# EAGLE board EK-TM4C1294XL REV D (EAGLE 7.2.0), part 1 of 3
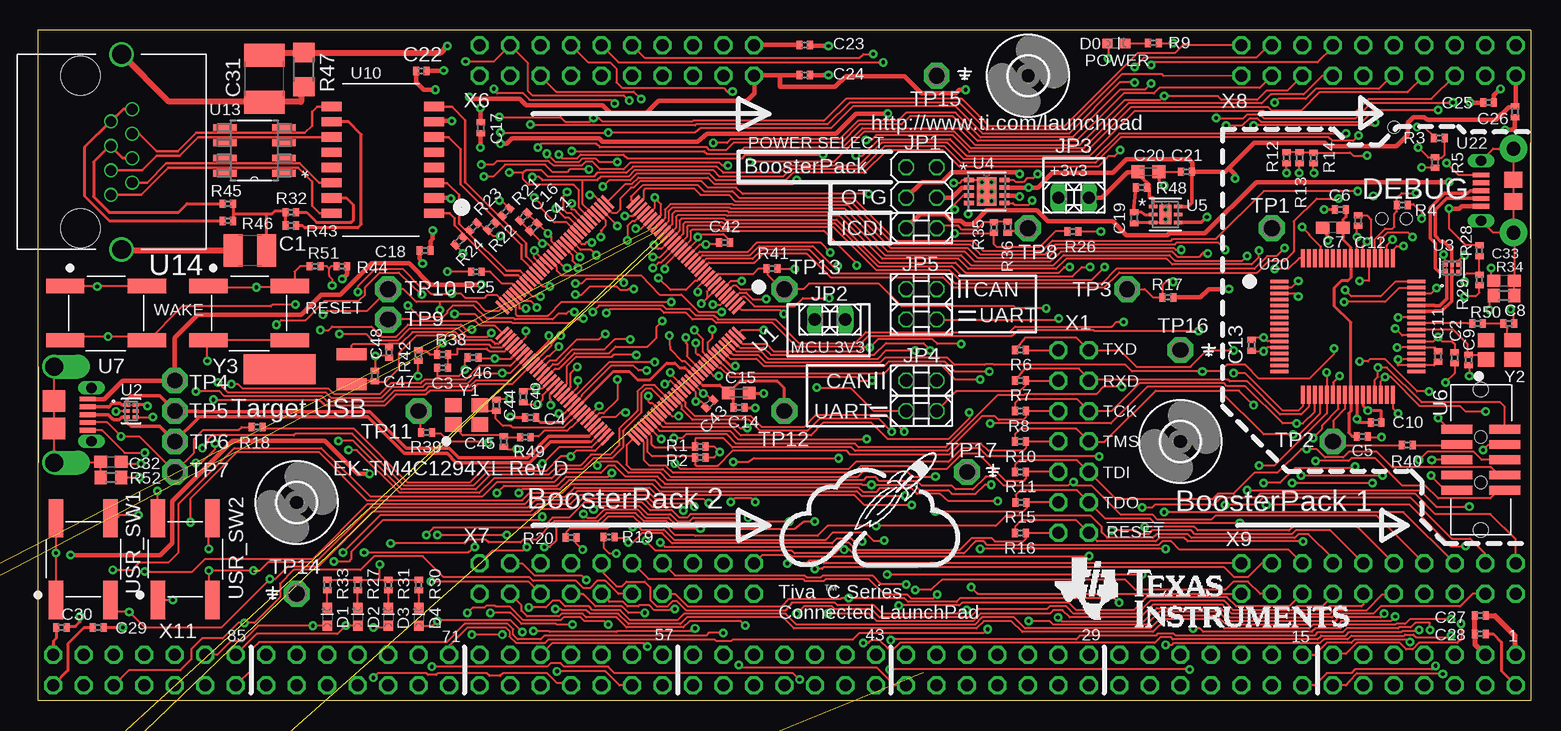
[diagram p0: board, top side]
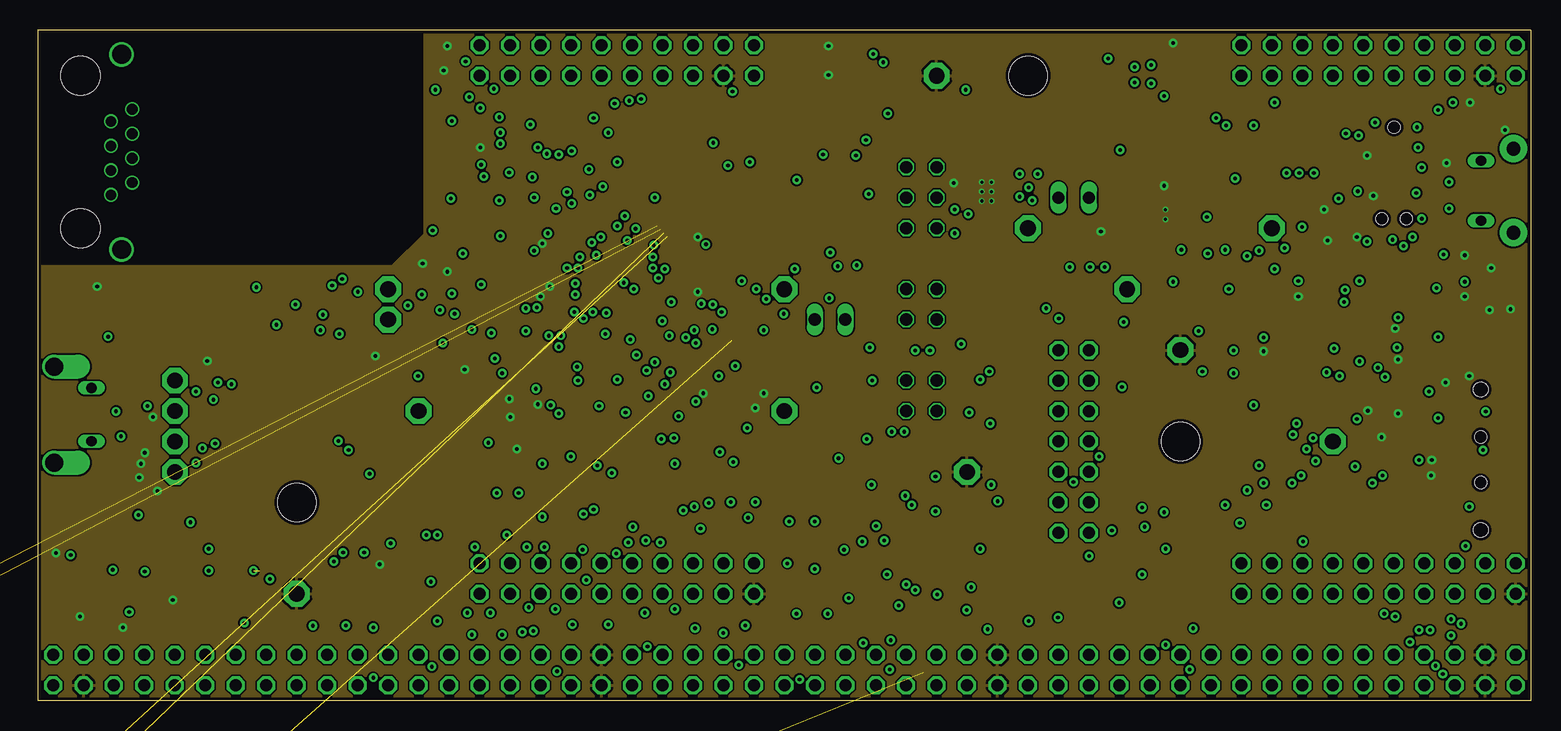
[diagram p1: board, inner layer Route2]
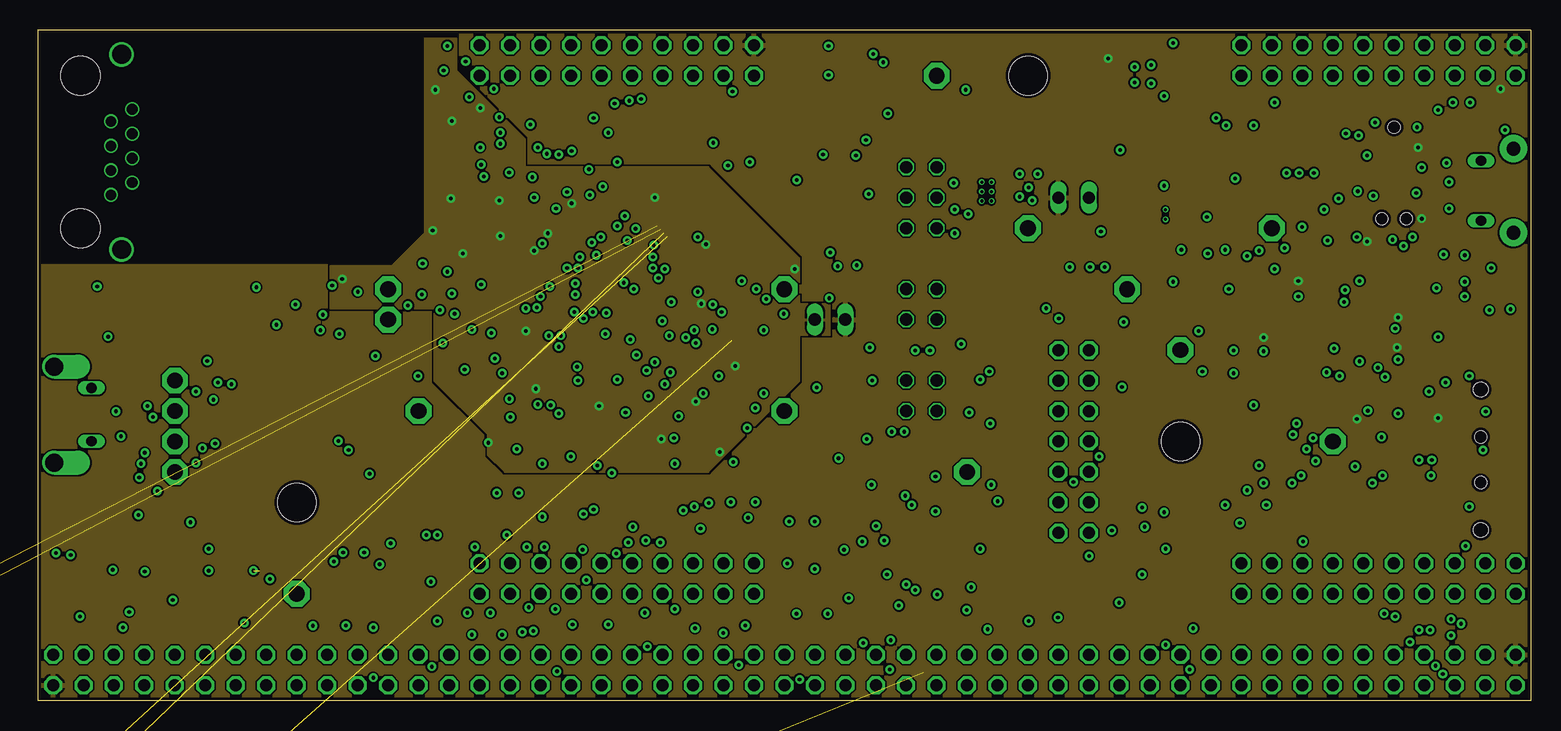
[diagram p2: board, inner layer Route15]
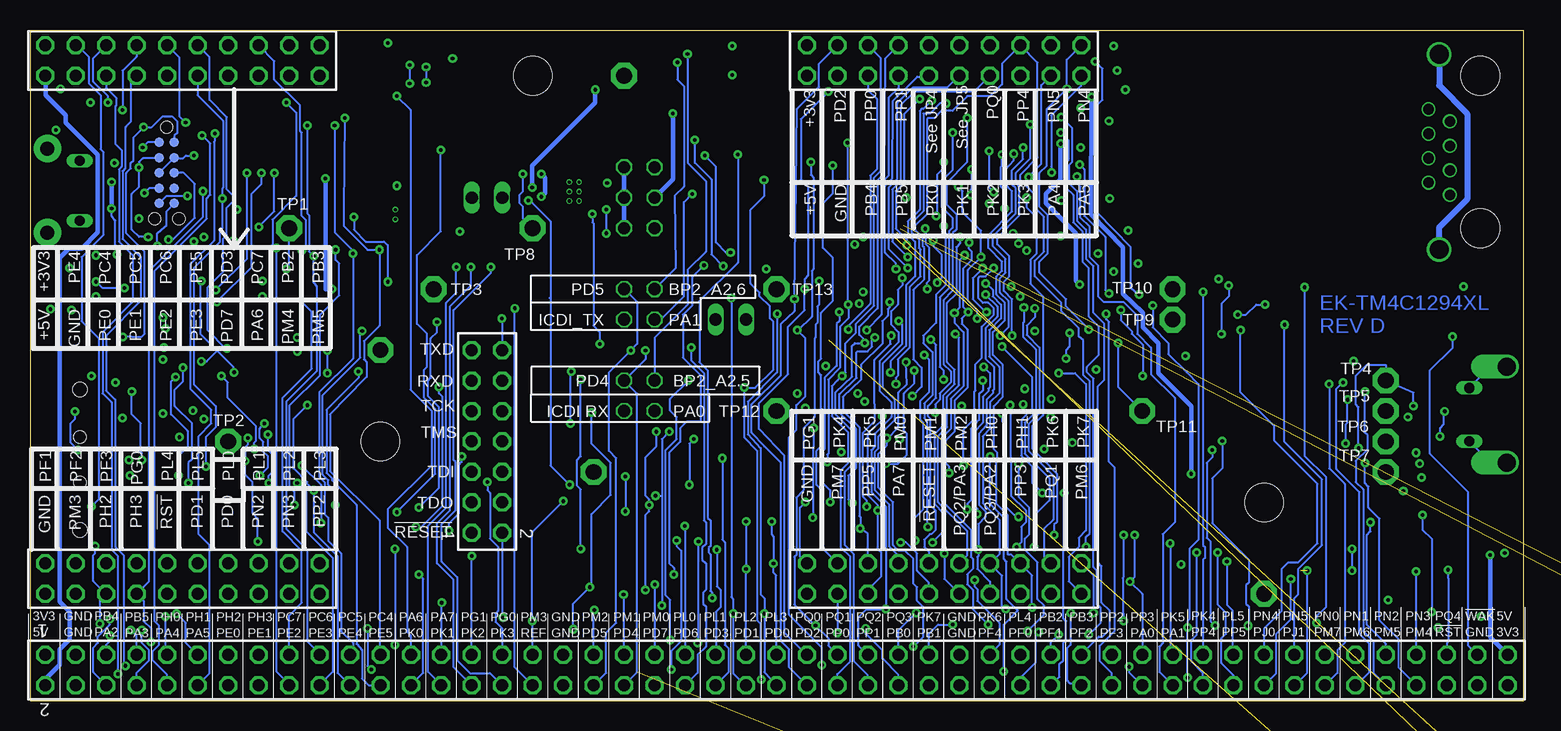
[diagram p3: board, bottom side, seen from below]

Size 124.46 x 55.88 mm. Coordinates in mm from the lower left corner, seen from the top.
Outline: 124.46,55.88 124.46,0 0,0 0,55.88 124.46,55.88
Copper layers (1+2*15+16): Top 0.035mm / dielectric 0.22mm / Route2 0.035mm / dielectric 1mm / Route15 0.035mm / dielectric 0.22mm / Bottom 0.035mm
Design rules "default *": minimum track width 6mil, minimum drill 12mil, track to track 6mil, track to pad 6mil, pad to pad 5mil, via to via 6mil, smd to smd 5mil, copper to edge 10mil, drill to drill 8mil, minimum pad ring 4mil, minimum via ring 8mil, stop-mask expansion 2mil, vias tented up to drill 13mil, thermal gap 8mil
Net classes: 1 USB: width 0.275 mm, clearance 0.152 mm; 2 Ethernet: width 0.22 mm, clearance 0.152 mm

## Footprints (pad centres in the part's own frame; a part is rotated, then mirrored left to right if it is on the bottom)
C1210 = smd 1.6 x 2.7: 1 -1.4,0; 2 1.4,0
C0402 = smd 0.5 x 0.7: 1 -0.45,0; 2 0.45,0
C0603 = smd 1.1 x 1: 1 -0.85,0; 2 0.85,0
C0603K = smd 1.05 x 1.08: 1 -0.875,0; 2 0.875,0
C1812 = smd 1.9 x 3.4: 1 -1.95,0; 2 1.95,0
CHIPLED_0603 = smd 0.8 x 0.8: A 0,-0.75; C 0,0.75
3,2 = hole 3.2: 0,0
2X03 = drill 1.016 octagon: 1 -2.54,-1.27; 2 -2.54,1.27; 3 0,-1.27; 4 0,1.27; 5 2.54,-1.27; 6 2.54,1.27
1X02 = drill 1.016 long: 1 -1.27,0; 2 1.27,0
2X02 = drill 1.016 octagon: 1 -1.27,-1.27; 2 -1.27,1.27; 3 1.27,-1.27; 4 1.27,1.27
R0402 = smd 0.5 x 0.7: 1 -0.45,0; 2 0.45,0
R0603 = smd 1 x 1.1: 1 -0.85,0; 2 0.85,0
R1206 = smd 1.6 x 1.803: 1 -1.422,0; 2 1.422,0
SWITCH_6MM_6MM_TE_CON_SMD = smd 1.2 x 3.2: P$1 4.521,6.807; P$2 4.521,0; P$3 0,6.807; P$4 0,0
P1-13 = drill 1.321 pad 2.159 octagon: TP 0,0
TQFP-128 = smd 1.45 x 0.25: P$1 0,0; P$2 0,-0.4; P$3 0,-0.8; P$4 0,-1.2; P$5 0,-1.6; P$6 0,-2; P$7 0,-2.4; P$8 0,-2.8; P$9 0,-3.2; P$10 0,-3.6; P$11 0,-4; P$12 0,-4.4; P$13 0,-4.8; P$14 0,-5.2; P$15 0,-5.6; P$16 0,-6; P$17 0,-6.4; P$18 0,-6.8; P$19 0,-7.2; P$20 0,-7.6; P$21 0,-8; P$22 0,-8.4; P$23 0,-8.8; P$24 0,-9.2; P$25 0,-9.6; P$26 0,-10; P$27 0,-10.4; P$28 0,-10.8; P$29 0,-11.2; P$30 0,-11.6; P$31 0,-12; P$32 0,-12.4; P$65 15.45,-12.4; P$66 15.45,-12; P$67 15.45,-11.6; P$68 15.45,-11.2; P$69 15.45,-10.8; P$70 15.45,-10.4; P$71 15.45,-10; P$72 15.45,-9.6; P$73 15.45,-9.2; P$74 15.45,-8.8; P$75 15.45,-8.4; P$76 15.45,-8; P$77 15.45,-7.6; P$78 15.45,-7.2; P$79 15.45,-6.8; P$80 15.45,-6.4; P$81 15.45,-6; P$82 15.45,-5.6; P$83 15.45,-5.2; P$84 15.45,-4.8; P$85 15.45,-4.4; P$86 15.45,-4; P$87 15.45,-3.6; P$88 15.45,-3.2; P$89 15.45,-2.8; P$90 15.45,-2.4; P$91 15.45,-2; P$92 15.45,-1.6; P$93 15.45,-1.2; P$94 15.45,-0.8; P$95 15.45,-0.4; P$96 15.45,0 | smd 0.25 x 1.45: P$33 1.525,-13.925; P$34 1.925,-13.925; P$35 2.325,-13.925; P$36 2.725,-13.925; P$37 3.125,-13.925; P$38 3.525,-13.925; P$39 3.925,-13.925; P$40 4.325,-13.925; P$41 4.725,-13.925; P$42 5.125,-13.925; P$43 5.525,-13.925; P$44 5.925,-13.925; P$45 6.325,-13.925; P$46 6.725,-13.925; P$47 7.125,-13.925; P$48 7.525,-13.925; P$49 7.925,-13.925; P$50 8.325,-13.925; P$51 8.725,-13.925; P$52 9.125,-13.925; P$53 9.525,-13.925; P$54 9.925,-13.925; P$55 10.325,-13.925; P$56 10.725,-13.925; P$57 11.125,-13.925; P$58 11.525,-13.925; P$59 11.925,-13.925; P$60 12.325,-13.925; P$61 12.725,-13.925; P$62 13.125,-13.925; P$63 13.525,-13.925; P$64 13.925,-13.925; P$97 13.925,1.525; P$98 13.525,1.525; P$99 13.125,1.525; P$100 12.725,1.525; P$101 12.325,1.525; P$102 11.925,1.525; P$103 11.525,1.525; P$104 11.125,1.525; P$105 10.725,1.525; P$106 10.325,1.525; P$107 9.925,1.525; P$108 9.525,1.525; P$109 9.125,1.525; P$110 8.725,1.525; P$111 8.325,1.525; P$112 7.925,1.525; P$113 7.525,1.525; P$114 7.125,1.525; P$115 6.725,1.525; P$116 6.325,1.525; P$117 5.925,1.525; P$118 5.525,1.525; P$119 5.125,1.525; P$120 4.725,1.525; P$121 4.325,1.525; P$122 3.925,1.525; P$123 3.525,1.525; P$124 3.125,1.525; P$125 2.725,1.525; P$126 2.325,1.525; P$127 1.925,1.525; P$128 1.525,1.525
DRY6 = smd 0.559 x 0.305: 1 -0.356,0.508 | smd 0.508 x 0.305: 2 -0.381,0; 3 -0.381,-0.508; 4 0.381,-0.508; 5 0.381,0; 6 0.381,0.508
DRB8_2P4X1P65 = smd 0.838 x 0.356: 1 -1.473,0.965; 2 -1.473,0.33; 3 -1.473,-0.33; 4 -1.473,-0.965; 5 1.473,-0.965; 6 1.473,-0.33; 7 1.473,0.33; 8 1.473,0.965 | smd 1.651 x 2.388: 9 0,0 | drill 0.254: V 0.406,0.787; V_2 -0.406,0; V_3 -0.406,-0.787; V_4 -0.406,0.787; V_5 0.406,-0.787; V_6 0.406,0
DRV6_1P6X1 = smd 0.711 x 0.305: 1 -1.041,0.66; 2 -1.041,0; 3 -1.041,-0.66; 4 1.041,-0.66; 5 1.041,0; 6 1.041,0.66 | smd 1.016 x 1.6: 7 0,0 | drill 0.254: V 0,-0.406; V_2 0,0.406
CON_2X5_50MIL = smd 0.74 x 2.6: P1 0,0; P2 0,4.008; P3 1.27,0; P4 1.27,4.008; P5 2.54,0; P6 2.54,4.008; P7 3.81,0; P8 3.81,4.008; P9 5.08,0; P10 5.08,4.008 | hole 1: 4.44,2; 0.64,2 | hole 1.2: 8.407,2; -3.327,2
CON_USB_MICRO_AB_HIROSE_ZX62D-AB-5P8 = smd 1.35 x 0.4: P1 2.8,1.3; P2 2.8,0.65; P3 2.8,0; P4 2.8,-0.65; P5 2.8,-1.3 | smd 1.9 x 1.8: P$1 0,-1.15; P$2 0,1.15 | drill 0.85 pad 1.092 long: P$3 3.125,2.225; P$4 3.125,-2.225 | drill 1.5 pad 2 offset: P$5 0,-4; P$6 0,4
DIL28-3 = drill 0.813 long: 1 -16.51,-3.81; 2 -13.97,-3.81; 3 -11.43,-3.81; 4 -8.89,-3.81; 5 -6.35,-3.81; 6 -3.81,-3.81; 7 -1.27,-3.81; 8 1.27,-3.81; 9 3.81,-3.81; 10 6.35,-3.81; 11 8.89,-3.81; 12 11.43,-3.81; 13 13.97,-3.81; 14 16.51,-3.81; 15 16.51,3.81; 16 13.97,3.81; 17 11.43,3.81; 18 8.89,3.81; 19 6.35,3.81; 20 3.81,3.81; 21 1.27,3.81; 22 -1.27,3.81; 23 -3.81,3.81; 24 -6.35,3.81; 25 -8.89,3.81; 26 -11.43,3.81; 27 -13.97,3.81; 28 -16.51,3.81
MAG_PULSE_HX1188FNL = smd 0.76 x 1.67: P$1 0,0; P$2 1.27,0; P$3 2.54,0; P$4 3.81,0; P$5 5.08,0; P$6 6.35,0; P$7 7.62,0; P$8 8.89,0; P$9 8.89,8.55; P$10 7.62,8.55; P$11 6.35,8.55; P$12 5.08,8.55; P$13 3.81,8.55; P$14 2.54,8.55; P$15 1.27,8.55; P$16 0,8.55
BLUETOOTH_SMD = smd 2 x 1: 1 0,0; 2 0,-1.5; 3 0,-3; 4 0,-4.5; 5 0,-6; 6 0,-7.5; 7 0,-9; 8 0,-10.5; 9 0,-12; 10 0,-13.5; 11 0,-15; 12 0,-16.5; 13 0,-18; 22 13,-18; 23 13,-16.5; 24 13,-15; 25 13,-13.5; 26 13,-12; 27 13,-10.5; 28 13,-9; 29 13,-7.5; 30 13,-6; 31 13,-4.5; 32 13,-3; 33 13,-1.5; 34 13,0 | smd 1 x 1.8: 14 1.25,-19.75; 15 2.75,-19.75; 16 4.25,-19.75; 17 5.75,-19.75; 18 7.25,-19.75; 19 8.75,-19.75; 20 10.25,-19.75; 21 11.75,-19.75
D8 = smd 1.981 x 0.559: 1 -2.464,1.905; 2 -2.464,0.635; 3 -2.464,-0.635; 4 -2.464,-1.905; 5 2.464,-1.905; 6 2.464,-0.635; 7 2.464,0.635; 8 2.464,1.905
RJ45_TE_CON_NOMAG_NOLED = drill 0.89: 1 9.93,2.54; 2 8.91,4.32; 3 7.89,2.54; 4 6.87,4.32; 5 5.85,2.54; 6 4.83,4.32; 7 3.81,2.54; 8 2.79,4.32 | drill 1.57: 9 -1.78,3.43; 10 14.48,3.43 | hole 3.25: 0,0; 12.7,0
LQFP-64-PM = smd 1.5 x 0.3: P$1 0,0; P$2 0,-0.5; P$3 0,-1; P$4 0,-1.5; P$5 0,-2; P$6 0,-2.5; P$7 0,-3; P$8 0,-3.5; P$9 0,-4; P$10 0,-4.5; P$11 0,-5; P$12 0,-5.5; P$13 0,-6; P$14 0,-6.5; P$15 0,-7; P$16 0,-7.5; P$33 11.4,-7.5; P$34 11.4,-7; P$35 11.4,-6.5; P$36 11.4,-6; P$37 11.4,-5.5; P$38 11.4,-5; P$39 11.4,-4.5; P$40 11.4,-4; P$41 11.4,-3.5; P$42 11.4,-3; P$43 11.4,-2.5; P$44 11.4,-2; P$45 11.4,-1.5; P$46 11.4,-1; P$47 11.4,-0.5; P$48 11.4,0 | smd 0.3 x 1.5: P$17 1.95,-9.45; P$18 2.45,-9.45; P$19 2.95,-9.45; P$20 3.45,-9.45; P$21 3.95,-9.45; P$22 4.45,-9.45; P$23 4.95,-9.45; P$24 5.45,-9.45; P$25 5.95,-9.45; P$26 6.45,-9.45; P$27 6.95,-9.45; P$28 7.45,-9.45; P$29 7.95,-9.45; P$30 8.45,-9.45; P$31 8.95,-9.45; P$32 9.45,-9.45; P$49 9.45,1.95; P$50 8.95,1.95; P$51 8.45,1.95; P$52 7.95,1.95; P$53 7.45,1.95; P$54 6.95,1.95; P$55 6.45,1.95; P$56 5.95,1.95; P$57 5.45,1.95; P$58 4.95,1.95; P$59 4.45,1.95; P$60 3.95,1.95; P$61 3.45,1.95; P$62 2.95,1.95; P$63 2.45,1.95; P$64 1.95,1.95
TC2030-MCP-NL = smd 0.787 x 0.787: 1 1.27,-0.635; 2 2.54,-0.635; 3 3.81,-0.635; 4 5.08,-0.635; 5 6.35,-0.635; 6 6.35,0.635; 7 5.08,0.635; 8 3.81,0.635; 9 2.54,0.635; 10 1.27,0.635 | hole 1: 0,0; 7.62,-1.016; 7.62,1.016
CON_USB_MICRO_B_FCI_10118194 = smd 1.35 x 0.4: P1 2.7,1.3; P2 2.7,0.65; P3 2.7,0; P4 2.7,-0.65; P5 2.7,-1.3 | smd 1.5 x 1.35: P6 0,0.9; P7 0,-0.9 | drill 0.85 long: P8 2.7,2.5; P9 2.7,-2.5 | drill 1.15 pad 2.286: P10 0,-3.5; P11 0,3.5
TSW-107-02-S-D = drill 1 pad 1.5 octagon: 1 7.62,-1.27; 2 7.62,1.27; 3 5.08,-1.27; 4 5.08,1.27; 5 2.54,-1.27; 6 2.54,1.27; 7 0,-1.27; 8 0,1.27; 9 -2.54,-1.27; 10 -2.54,1.27; 11 -5.08,-1.27; 12 -5.08,1.27; 13 -7.62,-1.27; 14 -7.62,1.27
TSW-110-02-S-D = drill 1 pad 1.5 octagon: 1 11.43,-1.27; 2 11.43,1.27; 3 8.89,-1.27; 4 8.89,1.27; 5 6.35,-1.27; 6 6.35,1.27; 7 3.81,-1.27; 8 3.81,1.27; 9 1.27,-1.27; 10 1.27,1.27; 11 -1.27,-1.27; 12 -1.27,1.27; 13 -3.81,-1.27; 14 -3.81,1.27; 15 -6.35,-1.27; 16 -6.35,1.27; 17 -8.89,-1.27; 18 -8.89,1.27; 19 -11.43,-1.27; 20 -11.43,1.27
TSW-149-02-S-D = drill 1 pad 1.5 octagon: 1 60.96,-1.27; 2 60.96,1.27; 3 58.42,-1.27; 4 58.42,1.27; 5 55.88,-1.27; 6 55.88,1.27; 7 53.34,-1.27; 8 53.34,1.27; 9 50.8,-1.27; 10 50.8,1.27; 11 48.26,-1.27; 12 48.26,1.27; 13 45.72,-1.27; 14 45.72,1.27; 15 43.18,-1.27; 16 43.18,1.27; 17 40.64,-1.27; 18 40.64,1.27; 19 38.1,-1.27; 20 38.1,1.27; 21 35.56,-1.27; 22 35.56,1.27; 23 33.02,-1.27; 24 33.02,1.27; 25 30.48,-1.27; 26 30.48,1.27; 27 27.94,-1.27; 28 27.94,1.27; 29 25.4,-1.27; 30 25.4,1.27; 31 22.86,-1.27; 32 22.86,1.27; 33 20.32,-1.27; 34 20.32,1.27; 35 17.78,-1.27; 36 17.78,1.27; 37 15.24,-1.27; 38 15.24,1.27; 39 12.7,-1.27; 40 12.7,1.27; 41 10.16,-1.27; 42 10.16,1.27; 43 7.62,-1.27; 44 7.62,1.27; 45 5.08,-1.27; 46 5.08,1.27; 47 2.54,-1.27; 48 2.54,1.27; 49 0,-1.27; 50 0,1.27; 51 -2.54,-1.27; 52 -2.54,1.27; 53 -5.08,-1.27; 54 -5.08,1.27; 55 -7.62,-1.27; 56 -7.62,1.27; 57 -10.16,-1.27; 58 -10.16,1.27; 59 -12.7,-1.27; 60 -12.7,1.27; 61 -15.24,-1.27; 62 -15.24,1.27; 63 -17.78,-1.27; 64 -17.78,1.27; 65 -20.32,-1.27; 66 -20.32,1.27; 67 -22.86,-1.27; 68 -22.86,1.27; 69 -25.4,-1.27; 70 -25.4,1.27; 71 -27.94,-1.27; 72 -27.94,1.27; 73 -30.48,-1.27; 74 -30.48,1.27; 75 -33.02,-1.27; 76 -33.02,1.27; 77 -35.56,-1.27; 78 -35.56,1.27; 79 -38.1,-1.27; 80 -38.1,1.27; 81 -40.64,-1.27; 82 -40.64,1.27; 83 -43.18,-1.27; 84 -43.18,1.27; 85 -45.72,-1.27; 86 -45.72,1.27; 87 -48.26,-1.27; 88 -48.26,1.27; 89 -50.8,-1.27; 90 -50.8,1.27; 91 -53.34,-1.27; 92 -53.34,1.27; 93 -55.88,-1.27; 94 -55.88,1.27; 95 -58.42,-1.27; 96 -58.42,1.27; 97 -60.96,-1.27; 98 -60.96,1.27
NDK3.2X2.5 = smd 1.4 x 1.2: P$1 0,0; P$2 2.2,0; P$3 2.2,1.6; P$4 0,1.6
CRYSTAL_32K_SMD = smd 2.5 x 1: P$1 0,1.25; P$2 0,-1.25 | smd 6 x 2.5: P$3 -6,0

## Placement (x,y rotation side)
C1  1000pF  [C1210]  17.68,37.49 180 top
C2  0.1uF  [C0402]  118.11,28.57 270 top
C3  0.1uF  [C0402]  33.76,27.74 180 top
C4  0.1uF  [C0402]  41.07,23.6 180 top
C5  0.1uF  [C0402]  110.41,22 0 top
C6  1.0uF  [C0402]  108.58,40.92 180 top
C7  2.2uF  [C0603]  107.95,39.42 180 top
C8  12pF  [C0402]  122.63,31.42 0 top
C9  12pF  [C0402]  119.25,28.37 270 top
C10  0.1uF  [C0402]  111.56,23.16 0 top
C11  0.1uF  [C0402]  116.71,28.68 270 top
C12  0.1uF  [C0402]  110.06,40.01 270 top
C13  0.1uF  [C0402]  101.17,29.62 270 top
C14  1.0uF  [C0402]  58.45,24.41 0 top
C15  2.2uF  [C0603K]  58.45,25.63 0 top
C16  0.1uF  [C0402]  40.49,40.31 225 top
C17  0.1uF  [C0402]  36.93,47.73 270 top
C18  0.1uF  [C0402]  32.28,37.49 180 top
C19  0.1uF  [C0402]  91.39,40.23 270 top
C20  2.2uF  [C0603K]  92.58,44.07 0 top
C21  0.1uF  [C0402]  95.76,44.07 180 top
C22  0.1uF  [C0402]  31.98,52.48 0 top
C23  0.1uF  [C0402]  63.93,54.64 0 top
C24  0.1uF  [C0402]  63.93,52.12 0 top
C25  0.1uF  [C0402]  120.93,49.83 180 top
C26  0.1uF  [C0402]  123.14,49.07 270 top
C27  0.1uF  [C0402]  120.24,7.09 180 top
C28  0.1uF  [C0402]  120.24,5.56 180 top
C29  0.1uF  [C0402]  5.03,6.1 0 top
C30  0.1uF  [C0402]  1.98,6.1 0 top
C31  4700pF  [C1812]  18.9,51.82 90 top
C32  3300pF  [C0603]  6.1,19.89 0 top
C33  3300pF  [C0603]  122.22,34.98 180 top
C40  0.1uF  [C0402]  40.46,25.32 270 top
C41  0.1uF  [C0402]  41.33,39.45 225 top
C42  0.1uF  [C0402]  57.25,38.18 0 top
C43  0.1uF  [C0402]  56.01,24.74 45 top
C44  12pF  [C0402]  38.23,24.61 90 top
C45  12pF  [C0402]  38.84,21.59 270 top
C46  0.1uF  [C0402]  36.3,28.6 180 top
C47  12pF  [C0402]  28.09,27.05 90 top
C48  12pF  [C0402]  29.29,29.01 270 top
D0  [CHIPLED_0603]  89.92,54.76 270 top
D1  [CHIPLED_0603]  24.13,6.99 0 top
D2  [CHIPLED_0603]  26.67,6.99 0 top
D3  [CHIPLED_0603]  29.21,6.99 0 top
D4  [CHIPLED_0603]  31.75,6.99 0 top
H1  MOUNT-HOLE3.2  [3,2]  95.25,21.59 0 top
H4  MOUNT-HOLE3.2  [3,2]  21.59,16.51 0 top
H6  MOUNT-HOLE3.2  [3,2]  82.55,52.07 0 top
J1  [JUMP]  73.66,39.37 90 top
J2  [JUMP]  73.66,24.13 90 top
J3  [JUMP]  86.36,41.91 90 top
J4  [JUMP]  73.66,26.67 90 top
J5  [JUMP]  73.66,31.75 90 top
J6  [JUMP]  73.66,34.29 90 top
J7  [JUMP]  66.04,31.75 90 top
JP1  [2X03]  73.66,41.91 270 top
JP2  [1X02]  66.04,31.75 180 top
JP3  [1X02]  86.36,41.91 0 top
JP4  [2X02]  73.66,25.4 90 top
JP5  [2X02]  73.66,33.02 90 top
R1  10k  [R0402]  55.22,21.18 180 top
R2  10k  [R0402]  55.22,20.24 180 top
R3  10k  [R0402]  116.84,46.89 0 top
R4  10k  [R0402]  113.74,41.3 180 top
R5  10k  [R0402]  116.48,44.83 270 top
R6  0  [R0402]  81.92,29.21 180 top
R7  0  [R0402]  81.92,26.67 180 top
R8  0  [R0402]  81.92,24.13 180 top
R9  330  [R0402]  92.99,54.81 180 top
R10  0  [R0402]  81.92,21.59 180 top
R11  0  [R0402]  81.92,19.05 180 top
R12  5.6k  [R0402]  104.09,45.24 90 top
R13  5.6k  [R0402]  105.18,45.24 90 top
R14  5.6k  [R0402]  106.35,45.21 90 top
R15  0  [R0402]  81.97,16.51 180 top
R16  0  [R0402]  81.92,13.97 180 top
R17  100k  [R0402]  94.21,33.6 180 top
R18  100  [R0402]  18.29,22.78 180 top
R19  0  [R0402]  47.62,13.61 0 top
R20  0  [R0402]  44.45,13.59 180 top
R21  49.9  [R0402]  39.01,40.72 225 top
R22  49.9  [R0402]  37.82,39.52 45 top
R23  49.4  [R0402]  36.3,39.47 225 top
R24  49.9  [R0402]  35.1,38.28 45 top
R25  4.87k 1%  [R0402]  36.55,35.74 180 top
R26  100k  [R0402]  86.28,39.09 0 top
R27  330  [R0402]  26.67,9.63 270 top
R28  5.6k  [R0402]  120.17,37.49 90 top
R29  10k  [R0402]  120.17,35.05 90 top
R30  330  [R0402]  31.75,9.63 270 top
R31  330  [R0402]  29.21,9.63 270 top
R32  75  [R0402]  21.11,40.69 0 top
R33  330  [R0402]  24.13,9.63 270 top
R34  1M  [R0603]  122.22,33.76 0 top
R35  10k  [R0402]  79.71,39.42 270 top
R36  100k  [R0402]  80.85,39.45 90 top
R38  51  [R0402]  33.76,28.83 0 top
R39  0  [R0402]  32.41,22.33 0 top
R40  0  [R0402]  114.17,21.29 0 top
R41  0  [R0402]  61.21,36.02 0 top
R42  1M  [R0402]  31.72,28.75 270 top
R43  75  [R0402]  21.11,39.57 0 top
R44  10k  [R0402]  25.35,36.2 180 top
R45  75  [R0402]  15.85,41.4 180 top
R46  75  [R0402]  15.85,39.98 180 top
R47  1M  [R1206]  22.17,52.58 270 top
R48  [R0402]  92,42.76 0 top
R49  2k  [R0402]  40.64,21.95 0 top
R50  2k  [R0402]  120.02,31.42 0 top
R51  100  [R0402]  23.13,36.2 0 top
R52  1M  [R0603]  6.1,18.59 180 top
RESET  SWITCH_TACTILE  [SWITCH_6MM_6MM_TE_CON_SMD]  14.22,34.54 270 top
TP1  TPPAD1-13  [P1-13]  102.87,39.37 270 top
TP2  TPPAD1-13  [P1-13]  107.95,21.59 0 top
TP3  TPPAD1-13  [P1-13]  90.81,34.29 180 top
TP4  TPPAD1-13  [P1-13]  11.43,26.67 90 top
TP5  TPPAD1-13  [P1-13]  11.43,24.13 270 top
TP6  TPPAD1-13  [P1-13]  11.43,21.59 90 top
TP7  TPPAD1-13  [P1-13]  11.43,19.05 270 top
TP8  TPPAD1-13  [P1-13]  82.55,39.37 180 top
TP9  TPPAD1-13  [P1-13]  29.21,31.75 0 top
TP10  TPPAD1-13  [P1-13]  29.21,34.29 0 top
TP11  TPPAD1-13  [P1-13]  31.75,24.13 0 top
TP12  TPPAD1-13  [P1-13]  62.23,24.13 0 top
TP13  TPPAD1-13  [P1-13]  62.23,34.29 0 top
TP14  TPPAD1-13  [P1-13]  21.59,8.89 0 top
TP15  TPPAD1-13  [P1-13]  74.93,52.07 0 top
TP16  TPPAD1-13  [P1-13]  95.25,29.21 0 top
TP17  TPPAD1-13  [P1-13]  77.47,19.05 0 top
U1  TM4C1294NCPDT  [TQFP-128]  58.42,32.77 225 top
U2  TPD4S012_DRY_6  [DRY6]  7.77,24.13 0 top
U3  TPD4S012_DRY_6  [DRY6]  117.88,36.04 90 top
U4  TPS2052B_DRB_8  [DRB8_2P4X1P65]  79.1,42.42 0 top
U5  TPS73733_DRV_6  [DRV6_1P6X1]  94,40.5 0 top
U6  JTAG_ARM_10PIN  [CON_2X5_50MIL]  118.29,22.61 270 top
U7  CON_USB_HIROSE_MICRO_AB_ZX62D_AB_5P8  [CON_USB_MICRO_AB_HIROSE_ZX62D-AB-5P8]  1.35,23.83 0 top
U8  ATMEGA328P_PDIP  [DIL28-3]  not placed on the board
U9  ATMEGA328P_PDIP  [DIL28-3]  not placed on the board
U10  MAG_PULSE_HX1188FNL  [MAG_PULSE_HX1188FNL]  33.05,40.61 90 top
U11  HC_05  [BLUETOOTH_SMD]  not placed on the board
U13  SLVU2.8-4  [D8]  18.06,45.85 180 top
U14  JACK_RJ45_NOMAG_NOLED_TECON  [RJ45_TE_CON_NOMAG_NOLED]  3.56,52.07 270 top
U20  TM4C123GH6PMI  [LQFP-64-PM]  103.5,34.92 0 top
U21  TC2050-NL-MCP-NL  [TC2030-MCP-NL]  113.06,47.78 270 bottom
U22  CON_USB_FCI_MICRO_B_10118194  [CON_USB_MICRO_B_FCI_10118194]  123.01,42.49 180 top
USR_SW1  SWITCH_TACTILE  [SWITCH_6MM_6MM_TE_CON_SMD]  1.52,8.38 0 top
USR_SW2  SWITCH_TACTILE  [SWITCH_6MM_6MM_TE_CON_SMD]  10.03,8.38 0 top
WAKE  SWITCH_TACTILE  [SWITCH_6MM_6MM_TE_CON_SMD]  2.29,34.54 270 top
X1  TSW-107-02-S-D  [TSW-107-02-S-D]  86.36,21.59 270 bottom
X6  TSW-110-02-S-D  [TSW-110-02-S-D]  48.26,53.34 180 bottom
X7  TSW-110-02-S-D  [TSW-110-02-S-D]  48.26,10.16 180 bottom
X8  TSW-110-02-S-D  [TSW-110-02-S-D]  111.76,53.34 180 bottom
X9  TSW-110-02-S-D  [TSW-110-02-S-D]  111.76,10.16 180 bottom
X11  TSW-149-02-S-D  [TSW-149-02-S-D]  62.23,2.54 180 bottom
Y1  25Mhz  [NDK3.2X2.5]  34.65,23.01 0 top
Y2  16M  [NDK3.2X2.5]  120.73,28.42 0 top
Y3  CRYATL_32K_SMD  [CRYSTAL_32K_SMD]  26.16,27.61 0 top

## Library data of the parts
C1 = EK-TM4C1294XL REV A; GNUM: G10-C1210-C102-ZCA
C2 = ek-tm4c129exl; GNUM: G10-C0402-C104-HBA; POPOP: OMIT
C3-C5 C10-C13 C16-C19 C21-C30 C40-C43 C46 = ek-tm4c129exl; GNUM: G10-C0402-C104-HBA
C6 C14 = ek-tm4c129exl; GNUM: G10-C0402-C105-GBB
C7 = ek-tm4c129exl; GNUM: G10-C0603-C225-HBB
C8 C9 C44 C45 C47 C48 = ek-tm4c129exl; GNUM: G10-C0402-C120-AAC
C15 C20 = ek-tm4c129exl; DIGIKEY_PARTNUM: 311-1451-2-ND; GNUM: G10-C0603-C225-HBB
C31 = ek-tm4c129exl; GNUM: G10-C1812-C472-ZBA
C32 C33 = EK-TM4C1294XL REV A; GNUM: G10-C0603-C332-ABA
D0 D1-D4 = ek-tm4c129exl; GNUM: G14-D0603-GR00-AAA
H1 H4 H6 = holes; GNUM: G30-62S04-A112-AAA; POPOP: OMIT
J1-J7 = jumper; GNUM: G72-100MI-JMPA-AAA
JP1 = pinhead; GNUM: G22-THVEU-2X3P-BAB
JP2 JP3 = pinhead; GNUM: G22-THVEU-002P-AAA
JP4 JP5 = pinhead; GNUM: G22-THVEU-002P-BAB
R1-R5 R29 R35 R44 = ek-tm4c129exl; GNUM: G11-R0402-1002-AAA
R6-R8 R10 R11 R15 R16 R19 R20 R39-R41 = ek-tm4c129exl; GNUM: G11-R0402-0000-AAA
R9 R27 R30 R31 R33 = ek-tm4c129exl; GNUM: G11-R0402-3300-AAA
R12-R14 = ek-tm4c129exl; GNUM: G11-R0402-5601-AAA; POPOP: OMIT
R17 R26 R36 = ek-tm4c129exl; GNUM: G11-R0402-1003-AAA
R18 R51 = ek-tm4c129exl; GNUM: G11-R0402-1000-AAA
R21-R24 = ek-tm4c129exl; GNUM: G11-R0402-49R9-ABA
R25 = ek-tm4c129exl; GNUM: G11-R0402-4871-ABA
R28 = ek-tm4c129exl; GNUM: G11-R0402-5601-AAA
R32 R43 R45 R46 = ek-tm4c129exl; GNUM: G11-R0402-75R0-AAA
R34 R52 = EK-TM4C1294XL REV A; GNUM: G11-R0603-R105-AAA
R38 = ek-tm4c129exl; GNUM: G11-R0402-51R0-AAA
R42 = ek-tm4c129exl; GNUM: G11-R0402-1004-AAA
R47 = EK-TM4C1294XL REV A; GNUM: G11-R1206-R105-CAA
R48 = ek-tm4c129exl; GNUM: G11-R0402-5232-ABA; POPOP: OMIT
R49 R50 = ek-tm4c129exl; GNUM: G11-R0402-R202-AAA
RESET USR_SW1 USR_SW2 WAKE = ek-tm4c129exl; GNUM: G21-4P6MM-B3S1-AAA
TP1-TP17 = ek-tm4c129exl; GNUM: G20-K5000-TP00-AAA; POPOP: OMIT
U1 = EK-TM4C1294XL REV A; GNUM: G50-QF128-C1294-ALH
U2 U3 = ek-tm4c129exl; DATASHEETURL: http://www.ti.com/lit/gpn/TPD4S012; DESCRIPTION: 4-Channel USB ESD Solution with Power Clamp; FAMILY_NAME: ESD Solution; GENERIC_PART_NUMBER: TPD4S012; GNUM: G57-SMDRY-S012-AAA; INDUSTRY_STD_PKG_TYPE: SON; MANUFACTURER: Texas Instruments; MANUFACTURER_PART_NUMBER: tpd4s012_dry_6; PACKAGE_DESIGNATOR: DRY; PIN_COUNT: 6; VENDOR: Texas Instruments
U4 = ek-tm4c129exl; DATASHEETURL: http://www.ti.com/lit/gpn/TPS2052B; DESCRIPTION: Current-Limited, Power-Distribution Switches; FAMILY_NAME: USB POWER SWITCH; GENERIC_PART_NUMBER: TPS2052B; GNUM: G57-08SON-2052-AAA; INDUSTRY_STD_PKG_TYPE: SON; MANUFACTURER: Texas Instruments; MANUFACTURER_PART_NUMBER: tps2052b_drb_8; PACKAGE_DESIGNATOR: DRB; PIN_COUNT: 8; VENDOR: Texas Instruments
U5 = ek-tm4c129exl; GNUM: G51-DRV06-T733-AAA
U6 = ek-tm4c129exl; GNUM: G22-SMVES-2X5A-BBC
U7 = ek-tm4c129exl; GNUM: G20-USBU-THAB-CEB
U8 U9 = SparkFun-DigitalIC
U10 = ek-tm4c129exl; GNUM: G12-SOI16-1TO1-ZZQ
U11 = SerialPortBluetooth
U13 = ek-tm4c129exl; GNUM: G14-SOIC8-SLVU-DAA
U14 = ek-tm4c129exl; GNUM: G20-8RJ45-ENET-AAA
U20 = ek-tm4c129exl; GNUM: G50-QFP64-F120-EGC
U21 = ek-tm4c129exl; POPOP: OMIT
U22 = ek-tm4c129exl; GNUM: G20-USBU-THB-CEB
X1 = ek-tm4c129exl; GNUM: G22-THVEU-2X7P-BAB; OC_FARNELL: unknown; OC_NEWARK: unknown; POPOP: OMIT
X6-X9 = ek-tm4c129exl; GNUM: G22-THSTK-2X10-BAC; OC_FARNELL: unknown; OC_NEWARK: unknown
X11 = con-samtec; GNUM1: G22-THRE-1x49-AAC; GNUM2: G22-THRA-1X49-AAC; OC_FARNELL: unknown; OC_NEWARK: unknown; POPOP: OMIT
Y1 = ek-tm4c129exl; GNUM: G15-32X25-2506-AAA
Y2 = ek-tm4c129exl; GNUM: G15-32X25-1606-AAA
Y3 = EK-TM4C1294XL REV A; GNUM: G15-CMR2T-3272-AAA

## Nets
!DEBUG_RESET_OUT: R16.2 U6.P10 U20.P$23 X1.1
!EXTERNAL_DEBUG: R40.1 TP2.TP U20.P$24
!HIB: TP9.TP U1.P$65
!TARGET_RESET: R16.1 R51.1 RESET.P$3 RESET.P$4 X1.2 X7.10 X9.10 X11.94
!TARGET_RESET_FILTERED: C46.1 R44.2 R51.2 U1.P$70
!WAKE: R42.2 TP10.TP U1.P$64 WAKE.P$1 WAKE.P$2 X11.95
+3V3: C10.1 C11.1 C12.1 C13.1 C23.1 C25.1 C27.1 C29.1 D0.A JP2.1 JP3.1 R3.2 R4.1 R5.1 U6.P1 U20.P$2 U20.P$11 U20.P$26 U20.P$37 U20.P$42 U20.P$54 U21.1 X6.1 X8.1 X11.1 X11.98
+5V: C21.1 C24.1 C26.1 C28.1 C30.1 R17.1 U4.7 U5.6 X6.2 X8.2 X11.2 X11.97
BP2_A2.5: JP4.4 X6.9
BP2_A2.6: JP5.4 X6.11
CHASSIS: C1.2 C31.1 R47.2 U14.9 U14.10
DEBUG_ACTIVE: TP1.TP U20.P$64
DEBUG_PC0/TCK/SWCLK: R8.2 U6.P4 U20.P$19 U20.P$30 X1.9
DEBUG_PC1/TMS/SWDIO: R10.2 U6.P2 U20.P$20 U20.P$29 X1.7
DEBUG_PC2/TDI: R11.2 U6.P8 U20.P$22 X1.5
DEBUG_PC3/TDO/SWO: R15.2 U6.P6 U20.P$21 U20.P$53 X1.3
DEBUG_VBUS: JP1.5 R28.2 U3.6 U22.P1
EN0RXI_N [Ethernet]: R21.2 U1.P$53 U10.P$8
EN0RXI_P [Ethernet]: R22.2 U1.P$54 U10.P$6
EN0TXO_N [Ethernet]: R23.2 U1.P$56 U10.P$3
EN0TXO_P [Ethernet]: R24.2 U1.P$57 U10.P$1
GND: C2.2 C3.2 C4.2 C5.2 C6.2 C7.2 C8.2 C9.2 C10.2 C11.2 C12.2 C13.2 C14.2 C15.2 C16.2 C17.2 C18.2 C19.2 C20.2 C21.2 C22.2 C23.2 C24.2 C25.2 C26.2 C27.2 C28.2 C29.2 C30.2 C31.2 C32.2 C33.2 C40.2 C41.2 C42.2 C43.2 C44.2 C45.2 C46.2 C47.2 C48.2 R9.1 R12.2 R13.2 R14.2 R25.2 R26.2 R27.1 R29.1 R30.1 R31.1 R33.1 R34.1 R47.1 R52.1 RESET.P$1 RESET.P$2 TP14.TP TP15.TP TP16.TP TP17.TP U1.P$10 U1.P$17 U1.P$48 U1.P$55 U1.P$58 U1.P$80 U1.P$114 U2.4 U3.4 U4.1 U4.9 U4.V U4.V_2 U4.V_3 U4.V_4 U4.V_5 U4.V_6 U5.3 U5.7 U5.V U5.V_2 U6.P5 U6.P9 U7.P5 U20.P$3 U20.P$12 U20.P$27 U20.P$32 U20.P$34 U20.P$35 U20.P$39 U20.P$55 U21.3 U21.5 U21.9 U22.P5 USR_SW1.P$3 USR_SW1.P$4 USR_SW2.P$3 USR_SW2.P$4 WAKE.P$3 WAKE.P$4 X6.4 X7.2 X8.4 X9.2 X11.3 X11.4 X11.35 X11.36 X11.61 X11.62 X11.96
ICDI_RESET: C2.1 R3.1 U20.P$38 U21.10
ICDI_TCK: R4.2 U20.P$52 U21.4
ICDI_TDI: U20.P$50 U21.8
ICDI_TDO: U20.P$49 U21.6
ICDI_TMS: R5.2 U20.P$51 U21.2
ICDI_USBD_N [USB]: U3.2 U20.P$43 U22.P2
ICDI_USBD_P [USB]: U3.1 U20.P$44 U22.P3
ICDI_VDDC: C5.1 C6.1 C7.1 U20.P$25 U20.P$56
JACK_RX_N [Ethernet]: U10.P$9 U13.4 U13.5 U14.6
JACK_RX_P [Ethernet]: U10.P$11 U13.3 U13.6 U14.3
JACK_TX_N [Ethernet]: U10.P$14 U13.2 U13.7 U14.2
JACK_TX_P [Ethernet]: U10.P$16 U13.1 U13.8 U14.1
MCU_3V3: C16.1 C17.1 C18.1 C22.1 C40.1 C41.1 C42.1 C43.1 JP2.2 R1.1 R2.1 R21.1 R22.1 R23.1 R24.1 R39.2 R41.2 R44.1 U1.P$7 U1.P$8 U1.P$16 U1.P$26 U1.P$28 U1.P$39 U1.P$47 U1.P$51 U1.P$52 U1.P$69 U1.P$79 U1.P$90 U1.P$101 U1.P$113 U1.P$122 U10.P$2 U10.P$7
N$1: C9.1 U20.P$40 Y2.P$1
N$2: C8.1 R50.2 Y2.P$3
N$3: D0.C R9.2
N$4: D4.C R30.2
N$5: D3.C R31.2
N$6: D1.C R33.2
N$7: R26.1 R35.2 U4.3
N$8: C32.1 R52.2 U7.P$1 U7.P$2 U7.P$3 U7.P$4 U7.P$5 U7.P$6
N$9: C19.1 R48.1 U5.2
N$10: R36.1 TP8.TP U4.8
N$11: C3.1 R38.2 U1.P$68
N$12: R40.2 U6.P3
N$13: C20.1 JP3.2 R48.2 U5.1
N$14: D2.C R27.2
N$15: R28.1 R29.2 U20.P$46
N$16: R49.2 U1.P$89
N$17: R50.1 U20.P$41
N$20: C33.1 R34.2 U22.P6 U22.P7 U22.P8 U22.P9 U22.P10 U22.P11
N$29: C45.1 R49.1 Y1.P$1
N$30: C47.1 U1.P$67 Y3.P$2
N$31: C44.1 U1.P$88 Y1.P$3
N$32: R32.2 U10.P$15
N$33: C48.1 U1.P$66 Y3.P$1
N$34: R43.2 U10.P$10
N$36: C1.1 R32.1 R43.1 R45.1 R46.1
N$44: R45.2 U14.4 U14.5
N$45: R46.2 U14.7 U14.8
PA0: JP4.2 U1.P$33 X11.74
PA1: JP5.2 U1.P$34 X11.76
PA2: R20.2 U1.P$35 X11.6
PA3: R19.2 U1.P$36 X11.8
PA4: U1.P$37 X6.18 X11.10
PA5: U1.P$38 X6.20 X11.12
PA6: U1.P$40 X8.16 X11.25
PA7: U1.P$41 X7.8 X11.27
PB0: R18.1 U1.P$95 X11.58
PB2: U1.P$91 X8.17 X11.67
PB3: U1.P$92 X8.19 X11.69
PB4: U1.P$121 X6.6 X11.5
PB5: U1.P$120 X6.8 X11.7
PC4: U1.P$25 U11.1 X8.5 X11.23
PC5: U1.P$24 U11.2 X8.7 X11.21
PC6: U1.P$23 U8.11 X8.9 X11.19
PC7: U1.P$22 U8.10 X8.15 X11.17
PD0: U1.P$1 X9.14 X11.50
PD1: U1.P$2 X9.12 X11.48
PD2: U1.P$3 X6.3 X11.52
PD3: U1.P$4 X8.13 X11.46
PD4: JP4.3 U1.P$125 U9.11 X11.40
PD5: JP5.3 U1.P$126 U9.10 X11.38
PD6: U1.P$127 U4.4 X11.44
PD7: U1.P$128 X8.14 X11.42
PE0: U1.P$15 X8.6 X11.14
PE1: U1.P$14 X8.8 X11.16
PE2: U1.P$13 X8.10 X11.18
PE3: U1.P$12 X8.12 X11.20
PE4: U1.P$123 X8.3 X11.22
PE5: U1.P$124 X8.11 X11.24
PF0: D4.A U1.P$42 X11.66
PF1: U1.P$43 X9.1 X11.68
PF2: U1.P$44 X9.3 X11.70
PF3: U1.P$45 X9.5 X11.72
PF4: D3.A U1.P$46 X11.64
PG0: U1.P$49 X9.7 X11.31
PG1: U1.P$50 X7.1 X11.29
PH0: U1.P$29 X7.13 X11.9
PH1: U1.P$30 X7.15 X11.11
PH2: U1.P$31 X9.6 X11.13
PH3: U1.P$32 X9.8 X11.15
PJ0: U1.P$116 USR_SW1.P$1 USR_SW1.P$2 X11.82
PJ1: U1.P$117 USR_SW2.P$1 USR_SW2.P$2 X11.84
PK0: U1.P$18 X6.10 X11.26
PK1: U1.P$19 X6.12 X11.28
PK2: U1.P$20 X6.14 X11.30
PK3: U1.P$21 X6.16 X11.32
PK4: U1.P$63 X7.3 X11.77
PK5: U1.P$62 X7.5 X11.75
PK6: U1.P$61 X7.17 X11.63
PK7: U1.P$60 X7.19 X11.59
PL0: U1.P$81 X9.13 X11.43
PL1: U1.P$82 X9.15 X11.45
PL2: U1.P$83 X9.17 X11.47
PL3: U1.P$84 X9.19 X11.49
PL4: U1.P$85 X9.9 X11.65
PL5: U1.P$86 X9.11 X11.79
PM0: U1.P$78 X7.7 X11.41
PM1: U1.P$77 X7.9 X11.39
PM2: U1.P$76 X7.11 X11.37
PM3: U1.P$75 X9.4 X11.33
PM4: U1.P$74 X8.18 X11.92
PM5: U1.P$73 X8.20 X11.90
PM6: U1.P$72 X7.20 X11.88
PM7: U1.P$71 X7.4 X11.86
PN0: D2.A U1.P$107 X11.85
PN1: D1.A U1.P$108 X11.87
PN2: U1.P$109 X9.16 X11.89
PN3: U1.P$110 X9.18 X11.91
PN4: U1.P$111 X6.19 X11.81
PN5: U1.P$112 X6.17 X11.83
PP0: U1.P$118 X6.5 X11.54
PP1: U1.P$119 X6.7 X11.56
PP2: U1.P$103 X9.20 X11.71
PP3: U1.P$104 X7.16 X11.73
PP4: U1.P$105 X6.15 X11.78
PP5: U1.P$106 X7.6 X11.80
PQ0: U1.P$5 X6.13 X11.51
PQ1: U1.P$6 X7.18 X11.53
PQ2: R19.1 U1.P$11 X7.12 X11.55
PQ3: R20.1 U1.P$27 X7.14 X11.57
PQ4: U1.P$102 U4.5 X11.93
RBIAS: R25.1 U1.P$59
TARGET_ID: R18.2 TP7.TP U2.2 U7.P4
TARGET_RXD: JP4.1 R7.1 X1.12
TARGET_TCK/SWCLK: R1.2 R8.1 U1.P$100 X1.10
TARGET_TDI: R11.1 U1.P$98 X1.6
TARGET_TDO/SWO: R15.1 U1.P$97 X1.4
TARGET_TMS/SWDIO: R2.2 R10.1 U1.P$99 X1.8
TARGET_TXD: JP5.1 R6.1 X1.14
TARGET_VBUS: JP1.3 TP4.TP U1.P$96 U2.6 U4.6 U7.P1 X11.60
TARGET_VDDC: C4.1 C14.1 C15.1 TP12.TP U1.P$87 U1.P$115
USBD_N [USB]: TP5.TP U1.P$93 U2.1 U7.P2
USBD_P [USB]: TP6.TP U1.P$94 U2.3 U7.P3
VBAT: R38.1 R39.1 R42.1 TP11.TP
VBUS: JP1.2 JP1.4 JP1.6 R35.1 R36.2 U4.2
VCP_RXD: R6.2 U20.P$17 X1.13
VCP_TXD: R7.2 U20.P$18 X1.11
VERSION_0: R12.1 U20.P$61
VERSION_1: R13.1 U20.P$47
VERSION_2: R14.1 U20.P$48
VREF+: R41.1 TP13.TP U1.P$9 X11.34
VREG_EN: R17.2 TP3.TP U5.4

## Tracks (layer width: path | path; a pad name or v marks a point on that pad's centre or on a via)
!DEBUG_RESET_OUT  (via drill 0.3)
  Top 0.152: U20.P$23 108.43,25.45 108.43,24.31 107.06,22.94 107.06,22.63 v106.3,21.87 | R16.2 81.46,13.95 81.46,14.48 81.49,14.51 81.99,15.01 86.59,15.01 X1.1 87.61,13.97 88.32,13.26 93.19,13.26 93.5,13.56 95.56,13.56 95.86,13.26 v105.46,13.26 | U6.P10 121.77,17.53 121.08,16.84 116.74,16.84 115.67,17.91 113.77,17.91 111.48,20.19 109.5,20.19 109.27,19.96 v106.53,19.96
  Bottom 0.152: v105.46,13.26 105.46,15.16 105.92,15.62 105.92,18.21 106.53,18.82 v106.53,19.96 106.53,21.11 106.3,21.34 v106.3,21.87
!EXTERNAL_DEBUG
  Top 0.152: U20.P$24 108.95,24.3 107.97,23.32 107.97,21.61 | 107.97,21.61 TP2.TP | 107.97,21.61 108.33,21.26 113.5,21.26 R40.1
!HIB
  Top 0.152: TP9.TP 29.34,31.77 31.01,31.77 31.17,31.62 36.5,31.62 36.88,31.24 38.1,31.24 38.12,31.22 U1.P$65
!TARGET_RESET  (via drill 0.3)
  Top 0.152: RESET.P$4 15.54,34.52 15.24,34.52 15.32,34.44 v18.21,34.44 | v18.21,34.44 18.25,34.48 19.62,34.48 20.01,34.78 | 20.01,34.78 RESET.P$3 | v51.89,13.18 52.27,12.8 66.45,12.8 66.83,13.18 67.59,13.18 68.2,12.57 76.89,12.57 77.88,13.56 79.48,13.56 79.78,13.26 82.14,13.26 82.37,13.49 82.37,13.79 R16.1 X1.2 | v85.04,6.93 85.34,6.63 92.2,6.63 93.27,7.7 98.6,7.7 99.36,6.93 105.31,6.93 105.61,7.24 107.75,7.24 108.05,7.54 110.8,7.54 112.09,8.84 112.98,8.84 X9.10 | X7.10 48.41,8.89 47.32,9.98 46.63,9.98 46.02,9.37 45.49,9.37 44.88,9.98 41.3,9.98 41,10.29 33.83,10.29 32.08,12.04 28.04,12.04 26.9,10.9 21.34,10.9 20.19,9.75 20.19,8.61 18.06,6.48 v17.22,6.48 16.69,6.48 15.39,5.18 13.72,5.18 12.8,4.27 12.8,3.43 11.89,2.52 7.59,2.52 X11.94 | v18.22,34.44 v18.21,34.44 | R51.1 21.87,36.2 21.41,35.74 21.41,34.98 21.38,34.86 21.38,34.4 21.79,34.82 20.01,34.78
  Bottom 0.152: v51.89,13.18 51.44,13.18 50.52,12.27 50.52,10.82 49.53,9.83 X7.10 | X1.2 85.09,6.99 v85.04,6.93 | v18.21,34.44 18.21,20.42 16.46,18.67 16.46,7.77 17.22,7.01 v17.22,6.48
!TARGET_RESET_FILTERED  (via drill 0.3)
  Top 0.152: 39.55,28.6 | C46.1 36.88,28.5 v38.1,28.5 39.45,28.5 39.55,28.6 | R44.2 24.46,36.2 24.31,36.04 24.31,35.97 | v24.54,34.59 24.54,35.13 24.31,35.36 24.31,35.42 24.31,35.97 | v25.15,30.56 27.36,30.56 27.89,30.02 30.02,30.02 31.01,31.01 35.05,31.01 35.74,30.33 37.49,30.33 v37.8,30.63 | 24.31,35.97 24.08,36.2 23.77,36.2 23.79,36.19 R51.2 | U1.P$70 39.55,28.6
  Bottom 0.152: v24.54,34.59 24.54,33.68 25.15,33.07 v25.15,30.56 | v37.8,30.63 37.8,29.52 38.1,29.21 v38.1,28.5
!WAKE  (via drill 0.3)
  Top 0.152: WAKE.P$2 2.9,30.33 4.88,30.32 v5.87,30.32 8.38,30.32 8.84,29.79 WAKE.P$1 9.02,30.28 9.07,29.87 12.04,32.84 19.43,32.84 19.58,32.99 v21.49,32.99 | 33.53,33.22 36.58,33.22 37.34,32.46 38.42,32.46 U1.P$64 | 33.53,33.22 31.55,33.22 30.48,34.29 TP10.TP 29.21,34.24 27.43,32.46 24.08,32.46 v23.77,32.16 | v33.53,32.54 33.53,33.22 | v31.7,27.05 31.73,27.08 R42.2
  Bottom 0.152: X11.95 4.57,4.57 4.57,17.37 7.77,20.57 7.77,27.51 5.87,29.41 v5.87,30.32 | v23.77,32.16 23.09,32.16 22.25,32.99 v21.49,32.99 | v33.53,32.54 33.53,31.7 32.61,30.79 32.61,30.56 31.7,29.64 v31.7,27.05
+3V3  (via drill 0.3)
  Top 0.152: D0.A 89.23,54.76 v89.23,53.49 | U20.P$42 114.53,31.93 v113.39,31.93 | U20.P$54 110.45,37.91 v110.8,38.25 111.18,38.63 111.18,40.08 110.87,40.39 110.19,40.39 110.19,40.31 110.22,40.43 C12.1 | v115.06,46.1 115.9,45.26 116.51,45.26 R5.1 116.5,45.25 117.03,45.25 117.27,45.49 117.27,46.79 117.2,46.86 R3.2 | v115.37,40.16 115.37,40.69 114.68,41.38 114.3,41.38 114.27,41.38 R4.1 | U20.P$2 104.53,34.42 v105.08,34.98 | 116.48,29.18 C11.1 116.42,29.43 U20.P$37 113.31,29.43 v113.31,29.41 | U20.P$11 102.51,29.93 v102.18,30.25 102.17,30.27 101.51,30.27 101.35,30.1 C13.1 | U6.P1 117.68,22.61 v116.74,23.55
  Top 0.254: C29.1 4.38,6.06 3.85,6.06 2.52,4.72 2.52,2.52 X11.98 | U20.P$26 109.95,23.85 v109.96,23.47 109.96,23.24 110.03,23.16 C10.1
  Top 0.381: C23.1 59.72,54.63 X6.1 | C25.1 121.38,50.44 v121.92,50.98
  Top 0.406: C27.1 121.46,7.09 123.14,5.41 123.14,3.81 123.11,3.95 X11.1
  Bottom 0.152: U21.1 114.66,46.51 v115.06,46.1 | v105.08,34.98 105,34.9 | v113.31,29.41 113.39,29.41 | v116.74,23.55 116.74,23.47
  Bottom 0.381: v121.92,50.98 121.92,51.05
  pour Route15 (rank 2): 32.26,55.88 124.46,55.88 124.46,0 0,0 0,36.2 29.51,36.2 32.26,38.91
+5V  (via drill 0.3)
  Top 0.254: C30.1 1.53,5.19 1.29,4.95 1.29,3.96 1.22,3.89 1.33,3.87 X11.97 | X11.2 122,2.46 122,4.88 121.31,5.56 C28.1
  Top 0.305: U5.6 95.88,41.16 95.86,41.15 96.21,41.5 C21.1
  Top 0.356: U4.7 v82.6,42.75
  Top 0.381: 123.17,52.07 X8.2 123.19,49.77 C26.1 122.87,49.45 122.61,49.45 121.54,48.39 115.82,48.39 115.59,48.62 114.68,48.62 114.22,48.16 114.22,47.17 113.23,46.18 107.59,46.18 107.29,46.48 101.42,46.48 99.29,44.35 | 99.29,44.35 99.01,44.07 C21.1 96.24,44.12 96.24,44.81 95.94,45.11 90.75,45.11 89.61,43.97 84.58,43.97 83.36,42.75 v82.6,42.75 | R17.1 96.93,33.6 97.61,34.29 v99.29,34.29 | v99.82,43.51 99.82,43.81 99.29,44.35 | v77.34,50.9 76.81,50.9 76.53,50.62 73.66,50.62 72.24,52.05 67.36,52.05 66.45,51.13 61.87,51.13 61.87,52.12 | v2.74,12.12 10.21,12.12 11.2,13.11 11.2,16.61 16.23,21.64 23.93,21.64 26.67,18.9 v27.66,18.9 | v35.97,50.29 36.12,50.14 40.16,50.14 40.69,49.61 47.09,49.61 47.7,49 50.75,49 51.74,49.99 59.13,49.99 59.74,50.6 59.74,52.02 X6.2 59.74,52.12 61.87,52.12 | C24.1 61.87,52.12
  Bottom 0.381: v99.29,34.29 99.82,34.29 v99.82,43.51 | v77.34,50.9 77.34,49.84 82.6,44.58 v82.6,42.75 | X11.97 2.74,5.28 v2.74,12.12 | v35.97,50.29 36.04,40.54 33.38,37.8 33.38,33.91 31.7,32.31 31.7,31.09 30.4,29.79 30.4,27.28 27.66,24.54 v27.66,18.9 | X11.2 123.19,1.78 122,2.97 122,4.27 121.16,5.11 121.16,7.39 122,8.23 122,36.88 121.23,37.64 120.17,37.64 118.8,39.01 118.8,45.49 121.46,48.16 121.46,48.77 123.14,50.44 123.14,52.02 X8.2
BP2_A2.5  (via drill 0.3)
  Top 0.152: X6.9 50.57,53.57 68.5,53.57 68.81,53.87 v69.65,53.87
  Bottom 0.152: v69.65,53.87 69.65,44.81 68.12,43.28 68.12,37.41 69.65,35.89 69.65,32.99 72.39,30.25 JP4.4
BP2_A2.6  (via drill 0.3)
  Top 0.152: X6.11 48.41,53.19 v70.48,53.19
  Bottom 0.152: v70.48,53.19 70.48,51.74 69.95,51.21 69.95,42.82 70.71,42.06 70.64,36.04 JP5.4
CHASSIS
  Top 0.508: C1.2 7.09,37.49 U14.10 | U14.9 10.93,49.91 17.91,49.91 C31.1 20.06,49.89 21.95,49.89 21.95,50.83 22.1,50.83 | R47.2 21.84,51.05 22.1,50.8 22.1,50.83 | 22.1,51.05 22.1,50.83
  Bottom 0.508: U14.9 6.99,51.26 4.65,48.92 4.65,41.76 7.01,39.4 7.01,37.61 U14.10
DEBUG_ACTIVE  (via drill 0.3)
  Top 0.152: v103.1,35.97 104.24,35.97 105.15,36.88 U20.P$64
  Bottom 0.152: v103.1,35.97 102.87,36.2 TP1.TP
DEBUG_PC0/TCK/SWCLK  (via drill 0.3)
  Top 0.152: U20.P$19 106.45,24.08 105.46,23.09 v104.93,23.09 103.78,23.09 100.66,26.21 99.14,26.21 98.91,26.44 91.82,26.44 89.51,24.13 X1.9 86.61,25.15 81.84,25.15 81.49,24.8 81.49,24.19 81.38,24.08 | R8.2 81.38,24.08 | 81.38,24 81.38,24.08 | v112.09,18.75 v105.31,18.75 | U20.P$30 111.95,26.61 v112.32,26.98 112.78,26.98 115.21,24.54 118.57,24.54 119.02,24.08 v120.7,24.08 | U6.P4 121.84,21.34 121.69,21.26 120.85,21.26 v120.47,20.88
  Bottom 0.152: v105.31,18.75 104.62,19.43 104.62,20.34 105,20.73 105,21.57 105.31,21.87 105.31,22.63 v104.93,23.09 | v112.09,18.75 112.09,20.42 111.33,21.11 111.33,22.48 112.7,23.85 112.7,26.59 v112.32,26.98 | v120.47,20.88 121.08,21.49 121.08,23.09 120.7,23.47 v120.7,24.08
DEBUG_PC1/TMS/SWDIO  (via drill 0.3)
  Top 0.152: U20.P$20 106.91,25.43 106.91,23.93 105.16,22.17 v104.62,22.17 102.18,22.17 98.53,25.83 93.19,25.83 88.92,21.57 87.94,21.57 87.86,21.64 X1.7 87.61,21.59 86.56,22.63 81.92,22.63 81.46,22.17 81.46,21.79 81.53,21.72 R10.2 | v104.55,18.14 v111.25,18.14 | U20.P$29 111.45,26.72 111.71,26.98 v111.71,27.74 112.47,27.74 115.37,24.84 121.92,24.84 122.3,24.46 U6.P2
  Bottom 0.152: v104.55,18.14 104.55,18.75 104.24,19.05 104.24,20.5 104.62,20.88 v104.62,22.17 | v111.25,18.14 111.25,19.81 110.95,20.12 110.95,23.09 112.39,24.54 112.39,25.91 111.71,26.59 v111.71,27.74
DEBUG_PC2/TDI  (via drill 0.3)
  Top 0.152: X1.5 87.63,19.13 | 107.9,25.42 U20.P$22 107.97,25.5 107.97,26.52 v108.51,27.05 | X1.5 86.64,20.04 82.26,20.04 81.84,20.04 81.46,19.66 81.46,19.13 R11.2 | X1.5 89.92,16.76 97.92,16.76 98.37,17.22 99.67,17.22 101.42,18.97 103.33,18.97 105.31,20.95 v105.77,20.95 106.6,20.95 107.29,20.27 108.81,20.27 109.27,20.73 111.63,20.73 112.93,19.43 121.16,19.43 121.79,18.8 U6.P8
  Bottom 0.152: v108.51,27.05 107.97,26.52 107.97,25.22 105.61,22.86 105.61,21.64 105.77,21.49 v105.77,20.95
DEBUG_PC3/TDO/SWO  (via drill 0.3)
  Top 0.152: X1.3 87.76,16.51 | X1.3 87.63,16.54 86.64,17.53 81.92,17.53 81.53,17.14 81.53,16.61 R15.2 | 88.06,16.46 X1.3 | 87.94,16.46 87.88,16.51 X1.3 | v101.8,19.58 103.1,19.58 107.45,23.94 U20.P$21 107.44,25.49 v107.44,27.36 | v100.2,14.78 93.12,14.78 92.73,15.16 88.98,15.16 X1.3 | U20.P$53 110.95,34.98 v110.19,34.98 | v115.98,25.76 114.99,25.76 112.32,28.42 111.02,28.42 110.87,28.27 v110.19,28.27 | U6.P6 120.37,20.07 119.71,20.73 115.82,20.73 v115.14,20.04
  Bottom 0.152: v101.8,19.58 100.2,17.98 v100.2,14.78 | v110.19,34.98 110.26,34.9 110.26,30.56 108.85,29.15 | 108.85,29.15 107.52,27.81 107.52,27.43 v107.44,27.36 | v110.19,28.27 109.73,28.27 108.85,29.15 | v115.14,20.04 115.14,20.65 115.21,20.73 115.21,23.09 115.98,23.85 v115.98,25.76
DEBUG_VBUS  (via drill 0.3)
  Top 0.152: U3.6 117.35,36.42 117.35,37.11 v117.2,37.19 | R28.2 120.13,38.1 120.02,37.95 119.02,37.95 117.65,39.32 v117.65,41
  Top 0.381: JP1.5 72.39,39.4 73.53,40.54 75.67,40.54 76.2,40.01 76.96,40.01 77.27,39.7 77.95,39.7 79.1,40.84 83.29,40.84 84.2,39.93 89.61,39.93 90.75,38.79 94.18,38.79 94.34,38.94 97.31,38.94 101.58,43.2 v117.65,43.2 | U22.P1 118.69,41.19 118.49,41 v117.65,41
  Bottom 0.152: v117.2,37.19 117.2,37.8 117.35,37.95 117.35,40.01 117.65,40.39 v117.65,41
  Bottom 0.381: v117.65,41 v117.65,43.2
EN0RXI_N
  Top 0.22: 38.56,40.24 40.7,38.1 40.7,37.01 U1.P$53 | 38.56,40.24 35.62,43.18 35.62,48.38 34.52,49.48 33.07,49.48 U10.P$8 | R21.2 38.61,40.24 38.56,40.24
EN0RXI_P
  Top 0.22: 38.3,39.98 40.33,37.95 40.33,36.82 U1.P$54 | 38.3,39.98 35.25,43.03 35.25,45.93 34.24,46.94 33.07,46.94 U10.P$6 | R22.2 38.3,39.92 38.3,39.98
EN0TXO_N
  Top 0.152: 40.98,35.03 40.21,35.8
  Top 0.22: 40.21,35.8 39.07,35.8 35.79,39.07 | 35.79,39.07 35.11,39.75 35.11,42.16 34.14,43.13 33.07,43.13 U10.P$3 | R23.2 35.82,39.07 35.79,39.07 | U1.P$56 40.98,35.03
EN0TXO_P
  Top 0.152: 40.71,34.77 40.05,35.42
  Top 0.22: 40.05,35.42 38.91,35.42 35.49,38.84 | 35.49,38.84 34.74,39.6 34.74,40.19 34.34,40.59 33.07,40.59 U10.P$1 | R24.2 35.49,38.74 35.49,38.84 | U1.P$57 40.71,34.77
GND  (via drill 0.3)
  Top 0.152: C43.2 56.08,25.15 55.63,25.6 v55.47,25.6 54.46,26.62 U1.P$114 | U4.1 79.1,43.38 U4.9 U4.V_2 78.64,42.42 78.64,43.2 78.64,43.36 77.04,43.36 76.81,43.13 v76.35,43.13 | U2.4 v9.6,23.62 | C48.2 29.25,28.49 29.34,28.42 29.03,28.73 v28.14,28.73 | v28.14,28.73 28.2,28.66 | C47.2 28.14,27.62 v28.14,28.73 | R26.2 v88.62,39.09 | C20.2 C21.2 | R9.1 93.6,54.74 93.57,54.79 94.56,54.79 94.64,54.81 v94.64,54.79 | R33.1 R27.1 28.5,10.08 | 28.5,10.08 R31.1 R30.1 | 28.5,10.08 v28.5,11.35 | 8.9,20.64 v8.91,20.65 7.24,20.65 5.36,22.52 U7.P5 | USR_SW1.P$4 v1.52,12.29 USR_SW1.P$3 | v14.12,28.3 14.12,29.99 RESET.P$2 21.64,30.02 | RESET.P$1 21.48,30.25 21.42,30.25 21.64,30.02 | 21.72,30.02 21.64,30.02 | C3.2 33.3,27.52 33.3,27.05 35.13,27.05 35.59,27.51 v35.59,27.58 35.59,28.42 35.65,28.35 C46.2 | C16.2 40.92,39.24 40.94,39.05 | R25.2 v34.14,35.74 | 103.52,33.91 U20.P$3 104.83,33.92 v105.08,33.68 | 119.23,27.93 C9.2 119.33,27.74 v119.33,27.05 | v118.95,33.68 119.86,33.68 120.17,33.98 R29.1 | U20.P$55 109.96,36.38 v109.96,38.63 109.96,39.47 C12.2 | 110.87,45.34 v110.8,45.41 109.65,45.41 109.41,45.66 R14.2 105.21,45.66 R13.2 R12.2 | U22.P5 118.44,43.79 v117.42,44.81 | U20.P$39 113.75,30.43 v113.16,31.01 | 40.94,39.05 41.11,39.05 v42.06,38.1 42.44,38.1 U1.P$48 | C44.2 38.26,25.15 v39.32,25.15 | C42.2 57.75,38.26 57.15,38.86 55.24,38.86 v55.02,38.63 55.02,38.41 U1.P$17 | C41.2 40.93,39.05 40.94,39.05 | U5.3 92.96,39.85 94,39.85 | U5.V U5.7 | C40.2 40.54,24.92 40.78,24.67 41.67,24.67 v41.68,24.69 42.06,25.07 42.06,25.46 U1.P$80 | C45.2 39.09,21.03 39.18,20.94 39.91,20.94 v39.93,20.95 | USR_SW2.P$4 v11.25,8.38
  Top 0.152: C8.2 123.05,31.56 123.05,32.32 v122.76,32.61 | U20.P$35 v113.39,28.43 v113.39,28.42 113.39,27.93 U20.P$34 116.41,27.93 C11.2 | C2.2 118.11,27.28 v117.35,26.52 | U20.P$32 112.95,24.36 v113.39,23.93 | U20.P$12 102.5,29.43 v102.18,29.11 101.31,29.11 C13.2 | C5.2 111.11,21.95 v112.01,21.95 | WAKE.P$4 v4.95,34.52 7.85,34.52 7.92,34.44 WAKE.P$3 | U6.P9 117.12,17.75 v116.13,18.75 | U6.P5 116.38,20.07 v116.2,20.04 | U1.P$58 41.21,33.68 v41.91,33.68 | U1.P$55 41.38,35.2 42.06,34.52 v42.67,34.52 | U1.P$10 55.02,34.45 v55.02,34.06 | R34.1 121.08,34.14 121.08,33.38 121.01,33.3 v121.01,32.54 | C33.2 121.16,35.14 v121.16,36.04 | C32.2 7.4,19.74 v8.61,19.74 | R52.1 v8.46,18.59 | USR_SW2.P$3 10.06,15.47 9.98,15.54 v9.98,17.45 | C31.2 17.52,54 | C19.2 91.31,39.78 91.67,39.78 91.59,39.74 C19.2
  Top 0.254: C19.2 91.56,39.81 91.44,39.7 91.59,39.85 92.95,39.85 U5.3 | C20.2 93.46,43.32 v93.88,42.9 | 94,39.85 U5.V | 78.64,43.2 U4.V_4 U4.V | U4.V_2 U4.V_6 U4.V_5 U4.V_3 | v39.4,23.62 39.57,23.6 C4.2 | C15.2 60.33,25.63 v60.5,25.6 | C14.2 59.72,24.41 59.74,24.38 59.78,24.42 59.78,24.34 59.82,24.31 v59.82,24.38 | C29.2 v7.09,6.1 | C30.2 2.67,6.17 3.12,6.17 3.5,6.55 v3.5,7.01 | C6.2 v107.21,40.92 | C7.2 107.52,38.7 v107.52,38.33 | U20.P$27 110.45,24.57 v110.87,24.16 111.98,24.16 111.98,23.2 111.94,23.16 C10.2 | U3.4 118.39,36.55 v118.95,37.11
  Top 0.381: C23.2 64.58,54.56 v65.91,54.56 | C24.2 v65.91,52.12 | C26.2 123.14,47.78 122.91,47.55 v122.3,47.55 | C25.2 v119.41,49.84 | C22.2 33.81,52.48 v33.83,52.5 | C18.2 31.84,36.81 v32.08,36.42 | C17.2 36.93,46.43 v36.88,46.1
  Top 0.406: X11.3 119.82,4.64 119.82,5.45 119.79,5.49 C28.2 C27.2
  Top 0.508: 17.52,54 R47.1 33.58,54 v34.14,54.56
  Bottom 0.152: v28.5,11.35 28.5,11.43 | v8.91,20.65 8.84,20.57 | v59.82,24.38 59.74,24.38 | U21.5 113.06,42.06 v111.33,42.06 | U21.9 U21.3 112.47,45.19 111.71,45.19 111.48,45.41 v110.8,45.41 | v113.16,31.01 113.23,30.94 | v105.08,33.68 105,33.76 | v113.39,28.42 113.46,28.42 | v117.35,26.52 117.42,26.59 | v113.39,23.93 113.46,23.93 | v112.01,21.95 111.94,21.95 | v41.91,33.68 41.83,33.68 | v42.67,34.52 | v8.61,19.74 8.53,19.74 | v8.46,18.59 8.38,18.59 | v9.98,17.45 9.98,17.53 | v34.14,54.56 34.06,54.56
  Bottom 0.254: v93.88,42.9 93.95,42.82 | v39.4,23.62 39.47,23.62 | v7.09,6.1 7.01,6.1 | v107.21,40.92 107.14,40.77 | v107.52,38.33 107.52,38.41 | v110.87,24.16 110.72,24.23 | v118.95,37.11 118.87,37.03
  Bottom 0.381: v65.91,54.56 65.84,54.56 | v65.91,52.12 65.84,52.12 | v119.41,49.84 119.48,49.84 | v33.83,52.5 33.76,52.5 | v32.08,36.42 32.16,36.35
  pour Route2: 0,36.2 29.51,36.2 32.26,38.91 32.26,55.88 124.46,55.88 124.46,0 0,0
ICDI_RESET  (via drill 0.3)
  Top 0.152: U20.P$38 115.14,29.95 116.36,29.95 v116.72,30.31 117.05,29.95 117.88,29.95 118.11,29.72 C2.1 | R3.1 116.36,47.02 115.59,47.78 v114.99,47.78
  Bottom 0.152: v116.72,30.31 115.96,30.31 115.15,30.31 114.91,30.56 114.91,37.41 116.43,38.94 116.43,43.97 116.05,44.35 116.05,44.81 115.82,45.03 115.82,46.94 v114.99,47.78 114.3,47.78 113.39,48.69 112.62,48.69 112.17,48.23 112.17,47.32 112.42,47.07 U21.10
ICDI_TCK  (via drill 0.3)
  Top 0.152: U20.P$52 111.45,38.45 112.32,39.32 112.93,39.32 113.08,39.47 113.08,40.54 113.29,40.77 R4.2 113.29,41.89 113.69,42.29 v114.91,42.29
  Bottom 0.152: U21.4 114.5,42.7 v114.91,42.29
ICDI_TDI  (via drill 0.3)
  Top 0.152: U20.P$50 112.45,37.93 v112.93,38.41
  Bottom 0.152: U21.8 111.63,43.97 111.1,43.43 110.72,43.05 110.72,40.23 112.55,38.41 v112.93,38.41
ICDI_TDO  (via drill 0.3)
  Top 0.152: U20.P$49 112.95,37.54 113.29,37.87 v113.84,37.87
  Bottom 0.152: v113.84,37.87 113.84,38.94 113.23,39.47 113.08,39.62 113.08,40.77 U21.6
ICDI_TMS  (via drill 0.3)
  Top 0.152: U20.P$51 111.95,38.42 112.55,39.01 114.22,39.01 v114.61,38.63 | v115.37,44.42 116.2,44.42 116.22,44.41 116.3,44.41 R5.2
  Bottom 0.152: U21.2 113.74,45.19 115.06,45.19 115.37,44.88 v115.37,44.42 115.37,42.82 115.98,42.22 115.98,39.24 115.37,38.63 v114.61,38.63
ICDI_USBD_N
  Top 0.275: U20.P$43 116.38,32.42 116.43,32.48 117.06,32.48 117.87,33.29 117.87,35.65 U3.2 | 117.87,35.68 U3.2 | U22.P2 119.18,41.84 119.18,41.85 117.44,41.85 116.5,40.91 116.5,38.72 116.97,38.25 117.2,38.25 117.88,37.57 U3.2
ICDI_USBD_P
  Top 0.275: U20.P$44 116.41,32.92 116.43,32.9 116.88,32.9 117.44,33.46 117.44,35.49 117.35,35.59 117.37,35.61 U3.1 117.32,35.74 116.81,35.74 116.51,36.04 116.51,38.1 116.07,38.55 116.07,41.08 117.26,42.28 119.18,42.28 119.39,42.49 U22.P3
ICDI_VDDC
  Top 0.254: C6.1 109.04,40.69 109.12,40.69 109.04,40.62 109.04,40.31 108.8,40.07 C7.1 108.81,39.1 108.81,38.41 109.45,37.76 U20.P$56 109.45,35.24 109.19,34.98 108.66,34.98 108.05,34.37 108.05,32.92 109.45,31.52 U20.P$25 109.45,24.11 109.27,23.93 109.27,22.33 109.58,22.02 109.88,22.02 C5.1
JACK_RX_N
  Top 0.22: U14.6 8.47,47.24 9.93,45.78 11.68,45.78 13.21,47.3 15.54,47.3 | 15.54,47.3 20.47,47.3 | 20.47,47.3 22.25,47.3 22.86,47.91 22.86,49.07 23.29,49.51 U10.P$9 | U13.5 15.6,47.35 15.54,47.3 | U13.4 20.52,47.35 20.47,47.3
JACK_RX_P
  Top 0.22: U14.3 8.71,44.18 9.93,45.41 11.84,45.41 13.36,46.93 15.62,46.93 | 15.62,46.93 20.55,46.93 | 20.55,46.93 24.46,46.93 U10.P$11 | U13.6 15.6,46.91 15.62,46.93 | U13.3 20.52,46.91 20.55,46.93
JACK_TX_N
  Top 0.22: U14.2 9.12,43.16 10.72,44.76 15.52,44.76 | 15.52,44.76 20.65,44.76 | 20.65,44.76 21.84,44.76 23.45,43.16 U10.P$14 | U13.2 20.65,45.21 20.65,44.76 | U13.7 15.52,45.21 15.52,44.76
JACK_TX_P
  Top 0.22: U14.1 8.62,42.14 10.87,44.39 15.57,44.39 | 15.57,44.39 20.62,44.39 | 20.62,44.39 21.69,44.39 22.86,43.22 22.86,41.25 23.5,40.62 U10.P$16 | U13.1 20.62,43.94 20.62,44.39 | U13.8 15.57,43.94 15.57,44.39
MCU_3V3  (via drill 0.3)
  Top 0.152: 55.83,24.41 55.32,24.92 v54.86,24.92 54.9,24.95 54.83,24.95 54.86,25.22 54.86,25.68 54.25,26.29 | 31.47,52.47 C22.1 | v38.56,38.71 37.95,38.71 37.49,39.17 R22.1 37.28,39.3 36.8,39.78 36.68,39.8 R23.1 | v35.43,37.26 35.43,37.34 34.9,37.87 R24.1 34.72,37.97 | C16.1 40.69,40.62 40.79,40.62 C41.1 41.83,39.62 v42.52,38.94 | 39.4,41.07 R21.1 39.24,41.07 38.63,41.68 v38.48,41.68 | 42.75,38.79 v42.52,38.94 | 32.92,22.1 R39.2 32.94,22.25 33.6,22.25 34.29,21.57 36.96,21.57 37.03,21.49 v37.57,21.49 | R2.1 55.67,20.27 56.39,20.27 v56.84,20.73 56.39,21.18 R1.1 | v51.97,21.79 U1.P$101 | 41.57,26.02 arc90 v41.53,25.98 | R41.2 61.91,35.97 v63.09,35.97 | v41.53,25.98 42.02,25.98 U1.P$79 | 41.27,25.98 v41.53,25.98 | 55.63,24.46 55.83,24.41 | 55.83,24.41 C43.1 | C42.1 56.6,38.02 v55.7,38.02 55.19,38.02 U1.P$16 | 42.75,38.94 v42.52,38.94 | C40.1 40.62,25.76 40.83,25.97 41.52,25.97 v41.53,25.98 | U1.P$113 54.25,26.29 | 54.33,26.29 54.25,26.29 | 44.5,41.38 v44.5,41.44 44.5,40.92 44.73,40.92 44.88,40.77 44.88,40.75 U1.P$39 | U1.P$28 51.44,41.05 v51.44,41.91 51.97,41.38 51.97,40.46 U1.P$26 | U1.P$8 55.78,34.08 55.78,33.53 | 55.78,33.53 v55.32,33.07 | U1.P$7 55.79,33.53 55.78,33.53 | U1.P$51 41.38,37.47 v41.38,37.49 41.38,36.91 U1.P$52 | U1.P$69 40.69,30.31 v40.69,30.79 | U1.P$90 46.64,24.38 v46.79,24.54 | U1.P$47 42.82,38.28 42.82,38.63 v42.52,38.94
  Top 0.254: U1.P$122 57.75,27.89 v58.14,27.89
  Top 0.381: C22.1 31.55,52.43 31.55,51.51 32.16,50.9 v33.15,50.9 | U10.P$7 33.05,48.31 v34.52,48.31 | U10.P$2 34.16,41.88 v34.44,41.83 | C18.1 32.73,38.3 32.92,38.48 32.92,39.01 32.93,39.15 v32.92,39.17 | R44.1 25.76,36.12 25.77,36.1 25.77,35.52 v25.38,35.13 | C17.1 36.93,49.33 v36.88,49.38
  Bottom 0.152: v63.09,35.97 63.02,35.97 | v55.7,38.02 55.63,37.95 | v44.5,41.44 44.5,41.45 | v40.69,30.79 40.69,30.71 | v46.79,24.54 46.71,24.38 | v56.84,20.73 56.77,20.8
  Bottom 0.381: v33.15,50.9 33.07,50.9 | v34.52,48.31 34.44,48.31 | v34.44,41.83 34.37,41.91 | v32.92,39.17 32.92,39.09 | v25.38,35.13 25.3,35.13 | v36.88,49.38 36.96,49.38
  pour Route15: 38.94,19.05 55.88,19.05 63.5,26.67 63.5,30.48 66.04,30.48 66.04,33.02 63.5,33.02 63.5,36.83 55.88,44.45 40.64,44.45 40.64,46.76 34.9,52.5 34.9,55.17 32.23,55.17 32.23,38.94 29.49,36.2 24.38,36.2 24.38,32.69 28.12,32.69 33.02,32.64 33.02,26.67 37.49,22.25 37.49,20.5
N$1
  Top 0.152: U20.P$40 114.92,30.94 117.96,30.94 119.18,29.72 119.18,28.95 C9.1 119.48,28.81 120.16,28.81 120.32,28.65 120.51,28.43 Y2.P$1
N$2
  Top 0.152: Y2.P$3 122.53,30.4 122.52,30.42 122.52,31.03 122.3,31.24 122,31.32 C8.1 R50.2
N$3
  Top 0.152: D0.C 92.42,54.76 R9.2
N$4
  Top 0.152: R30.2 D4.C
N$5
  Top 0.152: R31.2 D3.C
N$6
  Top 0.152: D1.C R33.2
N$7  (via drill 0.3)
  Top 0.152: U4.3 77.14,42.09 76.43,41.38 v76.43,40.92 | v76.43,38.94 79.64,38.94 R35.2 79.7,38.02 79.93,37.8 83.52,37.8 84.81,39.09 R26.1
  Bottom 0.152: v76.43,40.92 v76.43,38.94
N$8
  Top 0.152: 5.05,21.6 U7.P$4 | U7.P$6 U7.P$2 U7.P$1 U7.P$5 5.49,19.82 C32.1 R52.2
  Bottom 0.152: U7.P$3 2.7,27.82 U7.P$6 | U7.P$4 2.7,19.82 U7.P$5
N$9
  Top 0.152: 91.43,40.77 C19.1 | 92.96,40.46 U5.2
  Top 0.254: 92.96,40.46 92.35,40.46 92.05,40.69 91.73,40.69 C19.1
  Top 0.305: R48.1 91.35,40.78 91.36,40.77 C19.1
N$10  (via drill 0.3)
  Top 0.152: v83.36,43.89 82.98,43.51 82.45,43.51 82.14,43.2 81.53,43.2 81.38,43.36 80.59,43.36 U4.8 | TP8.TP 81.74,39.14 81.69,39.09 81,39.09 R36.1
  Bottom 0.152: TP8.TP 83.36,40.18 83.36,41.15 83.67,41.45 83.67,42.14 83.36,42.44 v83.36,43.89
N$11
  Top 0.152: C3.1 34.21,28.49 34.21,28.5 R38.2 34.39,28.83 34.44,28.88 34.98,28.88 34.98,29.34 37.41,29.34 37.64,29.11 38.92,29.11 U1.P$68
N$12
  Top 0.152: R40.2 118.62,21.29 U6.P3
N$13
  Top 0.305: 91.67,44.07 C20.1 92.05,43.73 92.05,43.59 92.65,42.99 R48.2 92.66,42.76 92.66,41.91 92.96,41.91 U5.1
  Top 0.381: 91.75,44.03 C20.1 91.68,44.04 90.83,44.04 88.7,41.91 JP3.2
N$14
  Top 0.152: D2.C R27.2
N$15  (via drill 0.3)
  Top 0.152: R29.2 120.17,36.84 R28.1 120.17,35.74 120.05,35.62 119.14,35.62 118.95,35.43 v118.95,34.9 | U20.P$46 116.14,33.92 v116.59,34.37
  Bottom 0.152: v116.59,34.37 118.42,34.37 v118.95,34.9
N$16
  Top 0.152: R49.2 41.15,21.87 41.29,22.01 41.75,22.01 42.22,22.48 44.12,22.48 44.42,22.78 44.48,22.78 U1.P$89
N$17
  Top 0.152: R50.1 119.21,31.43 U20.P$41
N$20
  Top 0.152: U22.P9 121.31,45.99 U22.P10 U22.P7 U22.P6 U22.P11 | U22.P11 121.31,38.99 U22.P8 | U22.P11 122.96,38.95 123.08,38.87 C33.1 R34.2
N$29
  Top 0.152: R49.1 39.09,21.95 38.94,22.1 38.98,22.1 C45.1 38.7,22.1 35.43,22.1 35.26,22.28 35.26,22.66 Y1.P$1
N$30
  Top 0.152: C47.1 28.19,26.52 28.32,26.54 28.17,26.54 28.42,26.52 | 28.42,26.52 28.96,26.52 30.1,27.66 30.1,28.96 31.55,30.4 34.59,30.4 35.36,29.64 37.64,29.64 37.87,29.41 38.68,29.41 38.68,29.43 U1.P$67 | 28.42,26.52 28.34,26.52 27.96,26.67 27.02,26.67 Y3.P$2
N$31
